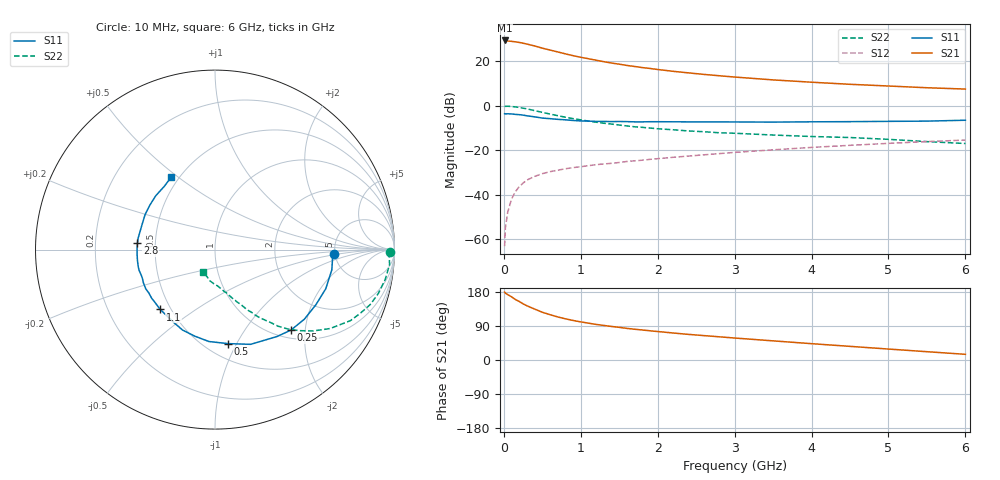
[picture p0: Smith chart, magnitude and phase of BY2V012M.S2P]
! SIEMENS Small Signal Semiconductors
! BFY420
! Si NPN RF SIEGET Grounded Emitter Transistor in MICRO-X
! VCE = 2 V  IC = 12 mA
! Common Emitter S-Parameters:  October  1996
# GHz  S  MA  R  50
!  f  S11  S21  S12  S22
! GHz  MAG  ANG  MAG  ANG  MAG  ANG  MAG  ANG
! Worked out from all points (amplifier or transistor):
!   36 points, 10 MHz to 6 GHz, reference 50 ohm
!   highest |S21| = 29.3 dB at 10 MHz (marker M1)
!   |S21| within 3 dB of that: start of sweep to 453.7 MHz
!   unconditionally stable (mu >= 1): 2.335 GHz to end of sweep
!   at 250 MHz: K = 0.21, MSG = 31.4 dB, |S12| = -34.8 dB
!   at 1.4 GHz: K = 0.80, MSG = 22.5 dB, |S12| = -25.9 dB
!   at 6 GHz: K = 1.09, MAG = 9.6 dB, |S12| = -15.4 dB
!   S11 on the Smith chart (normalised r, x): 10 MHz: 4.94, -0.39; 250 MHz: 1.16, -1.68; 500 MHz: 0.63, -0.92; 1.1 GHz: 0.44, -0.37; 2.8 GHz: 0.40, +0.04; 6 GHz: 0.45, +0.47
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0.01  0.6653 -1.9  29.34 179.2  0.0007 95.2  0.9752 -0.8
0.02  0.6567 -4.1  29.08 176.4  0.0018 86.6  0.9709 -1.7
0.1  0.6545 -19.5  28.07 166.8  0.008 82.0  0.9625 -10.1
0.15  0.6407 -28.6  27.27 159.6  0.0117 77.4  0.9419 -15.1
0.2  0.6311 -37.9  26.51 154.4  0.0152 75.5  0.9175 -19.5
0.25  0.6167 -46.6  25.45 148.3  0.0183 69.8  0.8828 -23.8
0.3  0.5951 -54.4  24.34 143.1  0.0214 66.3  0.8518 -27.7
0.4  0.5639 -69.4  22.09 134.4  0.0259 61.5  0.778 -34.4
0.5  0.5287 -82.2  19.7 126.0  0.0298 58.6  0.7111 -39.6
0.6  0.5132 -93.8  17.88 119.6  0.033 55.7  0.6512 -43.9
0.7  0.4953 -103.1  16.22 113.7  0.0357 54.0  0.5996 -47.5
0.8  0.4833 -111.9  14.67 108.7  0.0384 51.9  0.5532 -50.5
0.9  0.4672 -119.2  13.35 104.3  0.0408 51.7  0.514 -52.5
1.1  0.4522 -132.5  11.4 97.2  0.045 50.9  0.4528 -56.8
1.3  0.445 -142.4  9.79 91.2  0.0492 50.4  0.4052 -59.7
1.6  0.4401 -154.8  8.054 83.4  0.056 50.1  0.3519 -63.8
2.2  0.4362 -172.2  5.944 71.3  0.0695 49.3  0.289 -70.2
2.8  0.4338 175.1  4.725 61.2  0.0841 47.3  0.2475 -75.5
3.5  0.4295 161.7  3.812 50.5  0.1024 43.9  0.22 -81.4
4.5  0.4396 145.4  3.035 36.0  0.1291 37.0  0.1933 -90.9
5.5  0.4518 128.6  2.54 21.9  0.1569 28.6  0.1565 -106.8
6  0.473 120.9  2.373 15.0  0.1694 24.0  0.1419 -117.9
